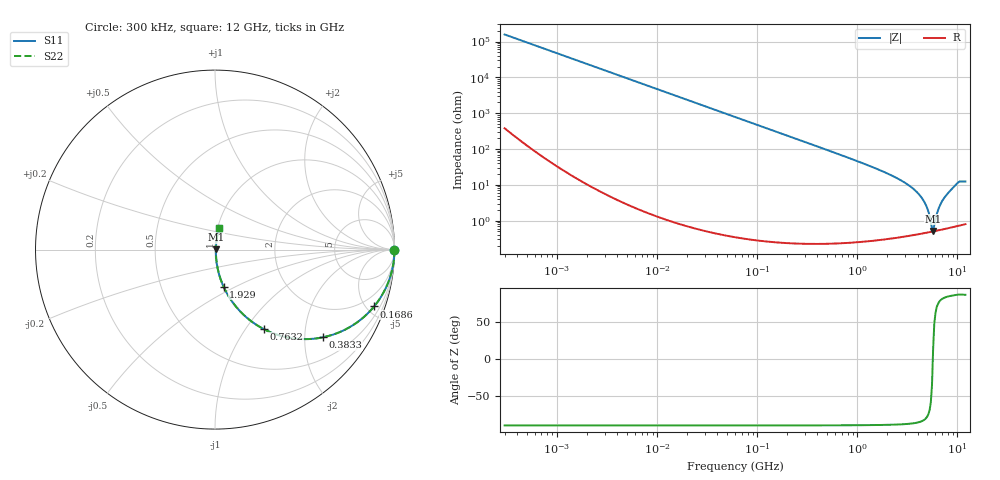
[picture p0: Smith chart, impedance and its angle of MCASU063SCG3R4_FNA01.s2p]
! MCASU063SCG3R4_FNA01  S-PARAMETER MODEL  ( General Type )
! Model Generated by TAIYO YUDEN Corporation (http://www.ty-top.com)
! Version 1.0
! TAIYO YUDEN Control No. 130801
! Copyright(c) 2013 TAIYO YUDEN CO.,LTD. All Rights Reserved.
! Product Description (link to TY-COMPAS)
! https://ds.yuden.co.jp/TYCOMPAS/or/detail?pn=MCASU063SCG3R4CFNA01&u=M
! Products Name : Multilayer Ceramic Capacitors
! Characteristics :
!  Capacitance : 3.4 pF , Rated Voltage : 50V , TCC : CG / C0G
!  Case Size : 0.6 x 0.3 / 0.024 x 0.012 [mm/inch] , Thickness : 0.3 / 0.012 [mm/inch]
!  (Conditions: Temperature = 25 degC , DC Bias Current/Voltage = 0A / 0V)
! External Node Assignments :
!  1  o---| |---o  2
! GND o---------o GND
! Frequency Range : 0.3MHz  -  12000MHz  [ 401 STEP ]
# MHz S RI R 50
! Freq[MHz].  S11 Real  S11 Imag  S21 Real  S21 Imag  S12 Real  S12 Imag  S22 Real  S22 Imag
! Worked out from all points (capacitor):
!   401 points, 300 kHz to 12 GHz, reference 50 ohm
!   read as one part in series: C = 3.37 pF near 316.3 kHz
!   lowest |Z| = 514 mohm at 5.715 GHz (marker M1)
!   series resonance near 5.678 GHz, so ESL is about 230 pH
!   S11 on the Smith chart (normalised r, x): 300 kHz: open; 168.6 MHz: 1.00, -5.60; 383.3 MHz: 1.00, -2.45; 763.2 MHz: 1.00, -1.21; 1.929 GHz: 1.01, -0.43; 12 GHz: 1.02, +0.25
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0.3  1 -0.000635  1.94e-06 0.000635  1.94e-06 0.000635  1 -0.000635
1.769972  1 -0.00375  1.58e-05 0.00375  1.58e-05 0.00375  1 -0.00375
10.44266  0.9995 -0.0221  0.000495 0.0221  0.000495 0.0221  0.9995 -0.0221
60  0.9841 -0.1251  0.0159 0.1251  0.0159 0.1251  0.9841 -0.1251
168.5979  0.8865 -0.3167  0.1135 0.3167  0.1135 0.3167  0.8865 -0.3167
353.9943  0.6381 -0.4797  0.3619 0.4797  0.3619 0.4797  0.6381 -0.4797
383.2761  0.6004 -0.4889  0.3996 0.4889  0.3996 0.4889  0.6004 -0.4889
763.2128  0.2704 -0.4422  0.7296 0.4422  0.7296 0.4422  0.2704 -0.4422
1197.383  0.1261 -0.3285  0.8739 0.3285  0.8739 0.3285  0.1261 -0.3285
1928.972  0.0474 -0.2057  0.9526 0.2057  0.9526 0.2057  0.0474 -0.2057
2088.533  0.0396 -0.1872  0.9604 0.1872  0.9604 0.1872  0.0396 -0.1872
3190.978  0.0137 -0.0996  0.9863 0.0996  0.9863 0.0996  0.0137 -0.0996
4158.869  0.00694 -0.0522  0.9931 0.0522  0.9931 0.0522  0.00694 -0.0522
4747.894  0.00539 -0.0298  0.9946 0.0298  0.9946 0.0298  0.00539 -0.0298
5006.236  0.00507 -0.021  0.9949 0.021  0.9949 0.021  0.00507 -0.021
5420.343  0.00489 -0.00784  0.9951 0.00784  0.9951 0.00784  0.00489 -0.00784
5715.274  0.00498 0.00117  0.995 -0.00117  0.995 -0.00117  0.00498 0.00117
5868.704  0.00508 0.00545  0.9949 -0.00545  0.9949 -0.00545  0.00508 0.00545
6524.734  0.00585 0.022  0.9941 -0.022  0.9941 -0.022  0.00585 0.022
7448.838  0.00775 0.0438  0.9923 -0.0438  0.9923 -0.0438  0.00775 0.0438
9968.853  0.0187 0.1074  0.9813 -0.1074  0.9813 -0.1074  0.0187 0.1074
12000  0.0226 0.1198  0.9774 -0.1198  0.9774 -0.1198  0.0226 0.1198
